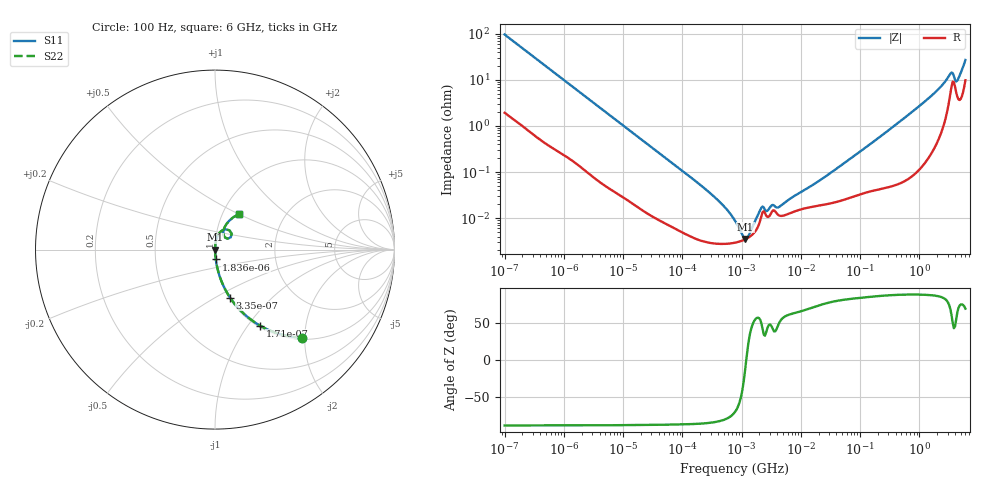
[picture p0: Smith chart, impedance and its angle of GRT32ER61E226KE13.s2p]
!Murata Part Number: GRT32ER61E226KE13
!These Parameters are Measured in Series Mode Connection
!Data Generated on Jun 19, 2026
!  o--ll--o
!Port1  Port2
!  o------o
!Operation Temp=25[degC], DC Bias Voltage=0[V]
!Freq. Start=100[Hz] Stop=6[GHz] 401[Steps]
# Hz S RI R 50
!Freq.(Hz) S11(Real) S11(Imag) S21(Real) S21(Imag) S12(Real) S12(Imag) S22(Real) S22(Imag)
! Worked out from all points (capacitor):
!   401 points, 100 Hz to 6 GHz, reference 50 ohm
!   read as one part in series: C = 16.3 uF near 109 Hz
!   lowest |Z| = 3.56 mohm at 1.159 MHz (marker M1)
!   series resonance near 1.201 MHz, so ESL is about 1.1 nH
!   S11 on the Smith chart (normalised r, x): 100 Hz: 1.04, -1.94; 171 Hz: 1.02, -1.14; 335 Hz: 1.01, -0.59; 1.836 kHz: 1.00, -0.11; 6 GHz: 1.20, +0.51
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100  0.4851 -0.4899  0.5149 0.4899  0.5149 0.4899  0.4851 -0.4899
171  0.2501 -0.423  0.7499 0.423  0.7499 0.423  0.2501 -0.423
335  0.0842 -0.2677  0.9158 0.2677  0.9158 0.2677  0.0842 -0.2677
717  0.0217 -0.1351  0.9783 0.1351  0.9783 0.1351  0.0217 -0.1351
1836  0.00435 -0.0546  0.9957 0.0546  0.9957 0.0546  0.00435 -0.0546
2008  0.00375 -0.0501  0.9963 0.0501  0.9963 0.0501  0.00375 -0.0501
40335  9.72e-05 -0.00262  0.9999 0.00262  0.9999 0.00262  9.72e-05 -0.00262
276587  2.96e-05 -0.000374  1 0.000374  1 0.000374  2.96e-05 -0.000374
774597  2.94e-05 -8.35e-05  1 8.35e-05  1 8.35e-05  2.94e-05 -8.35e-05
1159002  3.49e-05 -6.8e-06  1 6.8e-06  1 6.8e-06  3.49e-05 -6.8e-06
1658239  4.96e-05 6.56e-05  1 -6.56e-05  1 -6.56e-05  4.96e-05 6.56e-05
2268635  0.000136 0.000117  0.9999 -0.000117  0.9999 -0.000117  0.000136 0.000117
2713602  0.000107 9.61e-05  0.9999 -9.61e-05  0.9999 -9.61e-05  0.000107 9.61e-05
3245845  0.000137 0.000133  0.9999 -0.000133  0.9999 -0.000133  0.000137 0.000133
4246196  0.000116 0.00013  0.9999 -0.00013  0.9999 -0.00013  0.000116 0.00013
1.555665e7  0.000177 0.000486  0.9998 -0.000486  0.9998 -0.000486  0.000177 0.000486
3.124326e8  0.000545 0.00833  0.9995 -0.00833  0.9995 -0.00833  0.000545 0.00833
1.565993e9  0.00435 0.0438  0.9957 -0.0438  0.9957 -0.0438  0.00435 0.0438
2.679998e9  0.0197 0.0859  0.9803 -0.0859  0.9803 -0.0859  0.0197 0.0859
3.352442e9  0.0627 0.1126  0.9373 -0.1126  0.9373 -0.1126  0.0627 0.1126
4.385646e9  0.048 0.0794  0.952 -0.0794  0.952 -0.0794  0.048 0.0794
6e9  0.1356 0.1993  0.8644 -0.1993  0.8644 -0.1993  0.1356 0.1993
